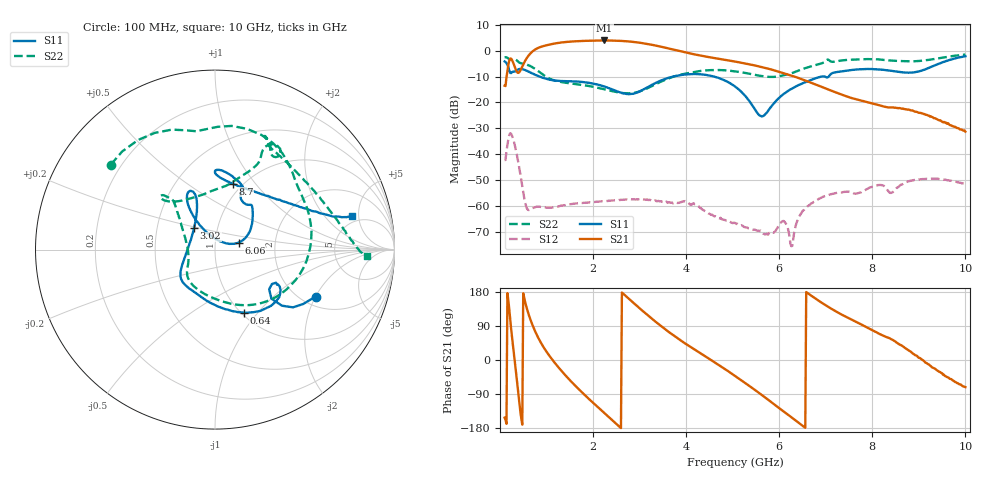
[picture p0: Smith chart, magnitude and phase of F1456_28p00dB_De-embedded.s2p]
! Integrated Device Technology
! Corporate Headquarters
! 6024 Silver Creek Valley Road
! San Jose, CA 95138  USA
! Phone:  1-408-284-8200
! Toll Free:  1-800-223-1366
! Webpage:  http://www.idt.com/
! Timing and RF Division
! 515 Groton Road, Suite 102
! Westford, MA 01886-6024
! Device:  F1456
! Description: 6-bit 0.5 dB Transmit Variable Gain Amplifier
! Frequency:  2100.0 -  2950.00 MHz
! Package:  6x6 mm Thin QFN Plastic Package: 28 pin
! State:  56
! Atten State:  28.0 dB
! Voltage:  +5.00 Volts
! Current:  216.967 mA
! Data:  The device was measured on a the F1455 evaluation board which has
!  individual transmission lines to the RF pins.  Data was collected
!  using a calibrated network analyzer.  The evaluation board was
!  de-embedded using a TRL calibration technique.
!  The reference plane is the edge of the package pin.
!  Pin  1 = CSb
!  Pin  2 = DATA
!  Pin  3 = CLK
!  Pin  4 = RSET
!  Pin  5 = GND
!  Pin  6 = RFIN  = Port 1
!  Pin  7 = GND
!  Pin  8 = NC
!  Pin  9 = NC
!  Pin 10 = NC
!  Pin 11 = NC
!  Pin 12 = NC
!  Pin 13 = NC
!  Pin 14 = /STBY
!  Pin 15 = GND
!  Pin 16 = RFOUT  = Port 2
!  Pin 17 = GND
!  Pin 18 = NC
!  Pin 19 = NC
!  Pin 20 = NC
!  Pin 21 = GND
!  Pin 22 = NC
!  Pin 23 = GND
!  Pin 24 = NC
!  Pin 25 = NC
!  Pin 26 = NC
!  Pin 27 = GND
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# GHz S dB R 50
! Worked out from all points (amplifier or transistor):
!   496 points, 100 MHz to 10 GHz, reference 50 ohm
!   highest |S21| = 4.0 dB at 2.24 GHz (marker M1)
!   |S21| within 3 dB of that: 807.6 MHz to 3.602 GHz (2.794 GHz wide, 127 % of centre)
!   unconditionally stable (mu >= 1): start of sweep to end of sweep
!   at 1.74 GHz: K = 254.10, MAG = 4.3 dB, |S12| = -58.9 dB
!   at 5.06 GHz: K = 1413.89, MAG = -3.2 dB, |S12| = -66.7 dB
!   at 10 GHz: K = 756.02, MAG = -21.7 dB, |S12| = -51.6 dB
!   S11 on the Smith chart (normalised r, x): 100 MHz: 2.37, -2.03; 640 MHz: 1.03, -0.85; 3.02 GHz: 0.77, +0.19; 6.06 GHz: 1.30, +0.10; 8.7 GHz: 0.90, +0.78; 10 GHz: 4.19, +4.12
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0.1  -4.11 -24.9  -13.52 -152.2  -42.30 50.3  -2.51 140.7
0.24  -8.62 -31.1  -3.04 82.5  -32.14 -77.6  -3.45 94.6
0.32  -8.01 -28.9  -6.25 -4.8  -36.61 -156.0  -3.23 68.0
0.42  -7.03 -36.5  -8.17 -118.4  -45.84 139.1  -4.60 40.5
0.52  -7.34 -50.8  -4.55 164.3  -56.84 118.0  -5.06 20.0
0.64  -8.27 -65.5  -1.28 111.8  -61.58 141.2  -5.79 -7.3
0.82  -9.76 -84.0  1.12 59.2  -60.38 119.8  -7.82 -45.3
1.14  -11.43 -110.6  2.71 -1.5  -60.68 85.2  -11.29 -90.9
1.76  -12.04 -139.0  3.82 -85.1  -58.93 50.5  -13.19 -133.1
2.24  -13.82 -154.4  4.02 -139.8  -58.17 33.4  -14.87 -147.8
2.62  -16.34 -179.9  3.83 178.1  -57.71 19.6  -16.33 -164.5
3.02  -15.55 134.4  3.09 134.4  -57.64 2.3  -15.56 165.3
3.4  -11.99 113.4  1.83 95.4  -58.11 -13.3  -12.48 142.6
4.12  -9.00 112.8  -1.17 32.6  -59.63 -48.5  -8.36 131.3
5.06  -13.93 122.8  -4.18 -42.7  -66.72 -97.9  -7.96 136.1
5.62  -25.38 66.2  -6.27 -91.8  -69.93 -173.6  -9.77 121.7
6.06  -17.20 16.5  -8.46 -132.7  -66.13 149.4  -9.61 91.5
6.26  -14.74 21.2  -9.60 -150.9  -75.65 141.4  -8.70 78.8
6.7  -11.17 40.7  -12.44 168.8  -59.04 143.8  -5.91 64.7
8.36  -7.62 88.6  -21.91 58.0  -54.73 57.5  -3.72 62.5
8.7  -8.40 74.9  -22.56 32.0  -51.12 66.8  -4.02 51.3
10  -2.09 13.8  -31.30 -71.5  -51.55 -27.1  -1.46 -2.6
